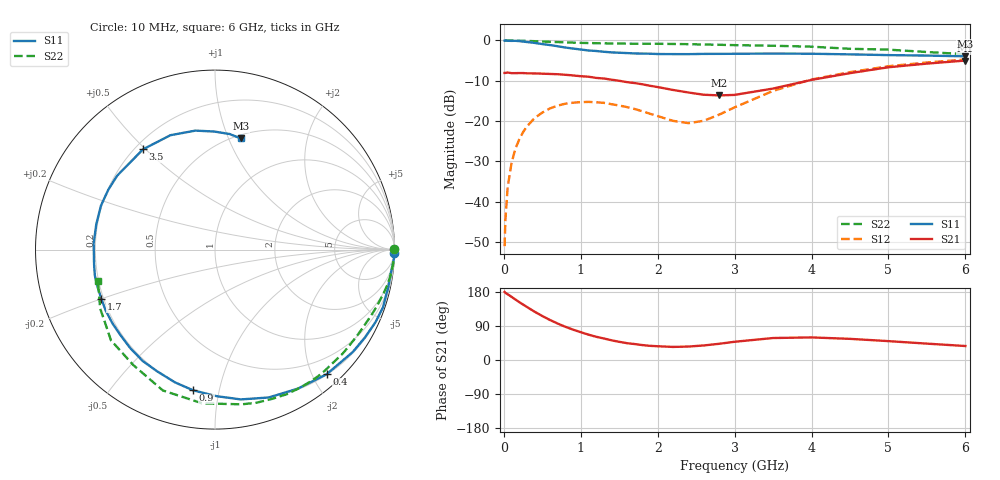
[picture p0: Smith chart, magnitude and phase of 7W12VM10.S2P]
! Infineon Technologies  Discrete & RF Semiconductors
! BFS17W
! Si NPN RF Bipolar Junction Transistor in SOT323
! VCE = 12 V  IC = 0.1 mA
! Common Emitter S-Parameters:  August  1999
# GHz  S  MA  R  50
!  f  S11  S21  S12  S22
! GHz  MAG  ANG  MAG  ANG  MAG  ANG  MAG  ANG
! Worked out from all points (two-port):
!   36 points, 10 MHz to 6 GHz, reference 50 ohm
!   highest |S21| = -4.99 dB at 6 GHz (marker M1); lowest = -13.6 dB at 2.8 GHz (marker M2)
!   |S21| within 3 dB of the highest: 41.48 MHz to 60.12 MHz (18.64 MHz wide, 36.7 % of centre); 4.542 GHz to end of sweep
!   lowest |S11| = -3.9 dB at 6 GHz (marker M3), VSWR 4.49, Z = 26.7 + j55.4 ohm
!   |S11| at or under -10 dB: nowhere
!   |S22| runs from -3.4 to 0.0 dB; largest |S21 - S12| = 0.4
!   S11 on the Smith chart (normalised r, x): 10 MHz: open; 400 MHz: 0.21, -2.22; 900 MHz: 0.20, -0.84; 1.7 GHz: 0.19, -0.20; 3.5 GHz: 0.23, +0.49; 6 GHz: 0.53, +1.11
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0.01  0.9947 -1.1  0.395 179.4  0.0028 86.3  0.9999 0.2
0.02  0.999 -2.6  0.395 177.3  0.0059 91.3  0.9953 -0.6
0.05  0.9905 -6.1  0.4 173.4  0.0152 87.1  0.9993 -1.5
0.1  0.9878 -12.0  0.393 166.7  0.0301 82.8  0.9999 -3.1
0.15  0.9896 -18.9  0.393 159.7  0.0453 77.8  0.9951 -4.6
0.2  0.9812 -24.4  0.394 152.9  0.0591 75.0  0.9933 -6.1
0.3  0.9564 -36.6  0.391 140.0  0.0856 67.3  0.9868 -9.0
0.4  0.9324 -48.1  0.39 127.4  0.1091 60.0  0.9793 -11.9
0.6  0.8767 -70.0  0.384 105.5  0.1434 47.7  0.9615 -17.1
0.9  0.7935 -98.8  0.368 80.1  0.1689 32.7  0.9391 -24.6
1.1  0.7509 -115.4  0.355 66.9  0.1728 25.1  0.9285 -29.4
1.4  0.7109 -137.5  0.326 52.0  0.1618 17.0  0.9191 -36.7
1.7  0.69 -156.5  0.296 42.1  0.1411 13.8  0.9107 -44.6
2.2  0.6769 177.1  0.243 34.5  0.1005 26.3  0.9045 -57.9
2.4  0.6764 167.8  0.226 35.5  0.0941 40.3  0.8995 -63.6
2.8  0.6817 150.6  0.208 42.8  0.1201 67.5  0.8838 -74.9
3.5  0.6878 125.6  0.253 58.0  0.2368 76.8  0.8596 -94.7
4  0.684 111.3  0.324 59.6  0.3281 70.7  0.8369 -110.3
4.5  0.6719 99.4  0.393 55.8  0.4045 62.5  0.788 -125.3
5  0.6579 90.4  0.465 49.8  0.4787 54.4  0.769 -138.9
5.5  0.6491 82.8  0.516 43.2  0.5331 46.3  0.7187 -152.9
6  0.6356 77.0  0.563 36.9  0.5799 39.0  0.6751 -165.2
